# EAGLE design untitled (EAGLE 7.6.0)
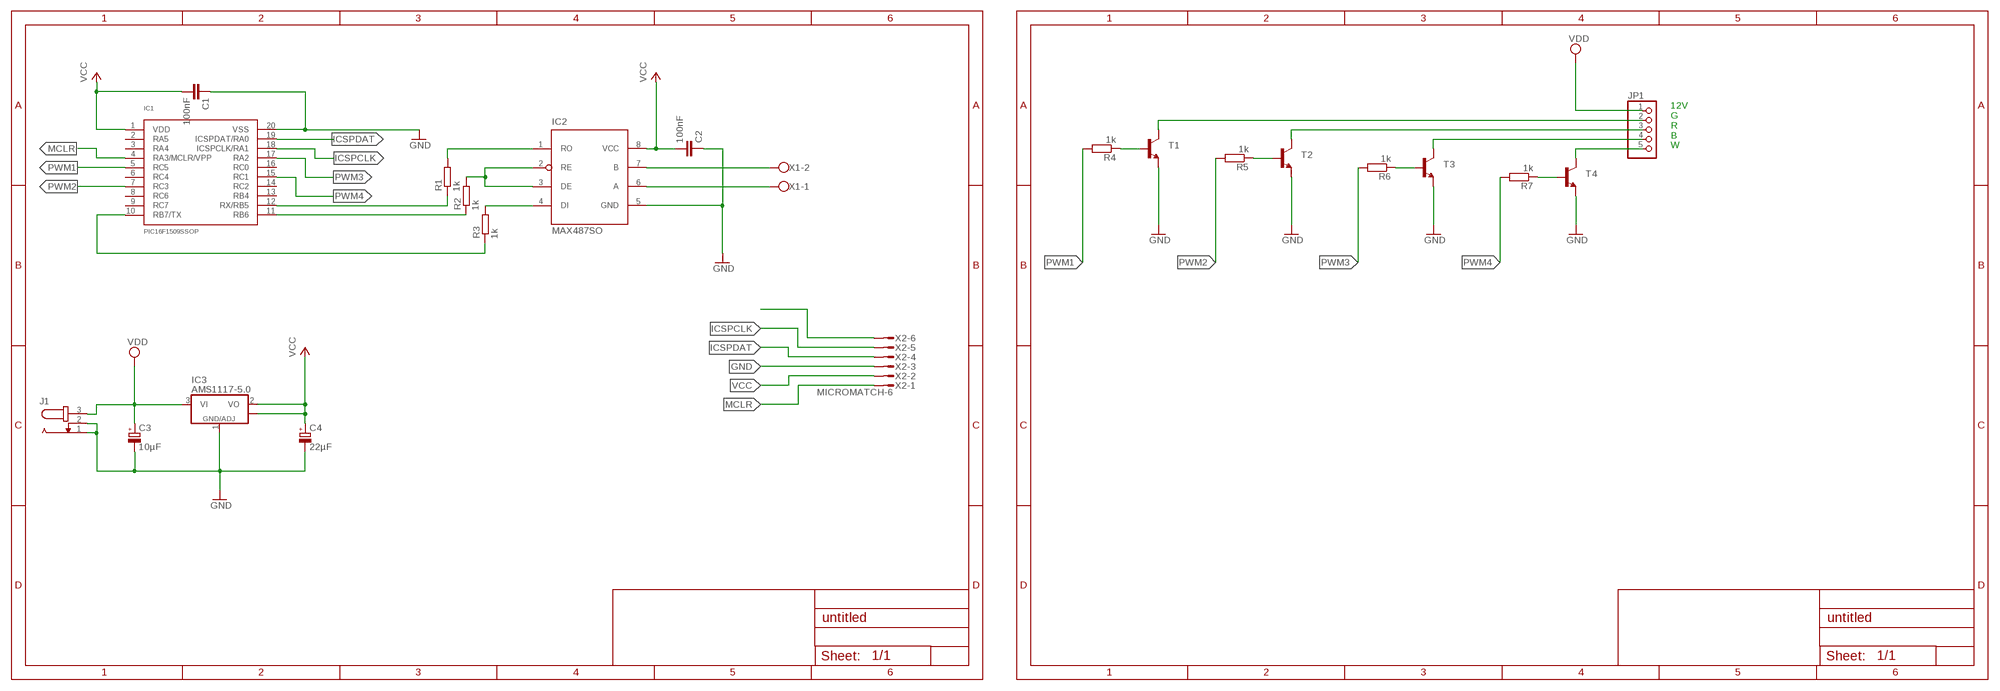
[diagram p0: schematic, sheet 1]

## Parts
C1  100nF  C-EUC0603  [C0603]
C2  100nF  C-EUC0603  [C0603]
C3  10µF  CPOL-EUF  [PANASONIC_F]
C4  22µF  CPOL-EUF  [PANASONIC_F]
IC1  PIC16F1509SSOP  [SSOP20]
IC2  MAX487SO  [SO08]
IC3  AMS1117-5.0  [SOT223]
J1  JACK-PLUG0  [SPC4077]
JP1  PINHD-1X5/90  [1X05/90]
R1  1k  R-EU_R0603  [R0603]
R2  1k  R-EU_R0603  [R0603]
R3  1k  R-EU_R0603  [R0603]
R4  1k  R-EU_R0603  [R0603]
R5  1k  R-EU_R0603  [R0603]
R6  1k  R-EU_R0603  [R0603]
R7  1k  R-EU_R0603  [R0603]
T1  -NPN-TO220V  [TO220V]
T2  -NPN-TO220V  [TO220V]
T3  -NPN-TO220V  [TO220V]
T4  -NPN-TO220V  [TO220V]
X1  W237-102  [W237-102]
X2  MICROMATCH-6  [MICROMATCH-6]

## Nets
GND: C1.1 C2.1 C3.- C4.- IC1.20(VSS) IC2.5(GND) IC3.1(GND/ADJ) J1.1 J1.2 T1.3(E) T2.3(E) T3.3(E) T4.3(E) X2.3
ICSPCLK: IC1.18(ICSPCLK/RA1) X2.5
ICSPDAT: IC1.19(ICSPDAT/RA0) X2.4
MCLR: IC1.4(RA3/MCLR/VPP) X2.1
N$1: JP1.2 T1.2(C)
N$2: IC1.10(RB7/TX) R3.1
N$3: IC2.2(RE) IC2.3(DE) R2.2
N$4: IC2.1(RO) R1.2
N$5: JP1.3 T2.2(C)
N$6: IC1.11(RB6) R2.1
N$7: IC1.12(RX/RB5) R1.1
N$8: IC2.4(DI) R3.2
N$9: JP1.4 T3.2(C)
N$10: JP1.5 T4.2(C)
N$11: IC2.7(B) X1.2
N$12: IC2.6(A) X1.1
N$13: R4.1 T1.1(B)
N$14: R5.1 T2.1(B)
N$15: R6.1 T3.1(B)
N$16: R7.1 T4.1(B)
N$22: X2.6
PWM1: IC1.5(RC5) R4.2
PWM2: IC1.7(RC3) R5.2
PWM3: IC1.17(RA2) R6.2
PWM4: IC1.15(RC1) R7.2
VCC: C1.2 C2.2 C4.+ IC1.1(VDD) IC2.8(VCC) IC3.2(VO) IC3.4(VO$1) X2.2
VDD: C3.+ IC3.3(VI) J1.3 JP1.1
Unconnected: IC1.2(RA5) IC1.3(RA4) IC1.6(RC4) IC1.8(RC6) IC1.9(RC7) IC1.13(RB4) IC1.14(RC2) IC1.16(RC0)

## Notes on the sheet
- 12V
  G
  R
  B
  W

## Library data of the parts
C1 C2 = rcl:C-EU: CAPACITOR, European symbol
C3 C4 = rcl:CPOL-EU: POLARIZED CAPACITOR, European symbol
IC1 = PIC16F:PIC16F1509: PIC16F1509 Flash: 14 KB RAM: 512 Byte Interner Oszillator: 16 MHz AD-Wandler: 12x 10-bit Schnittstellen: 1x UART, 1x SPI, 1x I2C Timer: 2x 8-bit, 1x 16-bit Besonderheiten: 4x 10-bit Standard-PWM
IC2 = maxim:MAX487
IC3 = AMS1117:AMS1117: Spannungsregler 1A
J1 = con-jack:JACK-PLUG: DC POWER JACK Power Jack, DC, Right Angle, Through Hole, Rated 5A at 16VDC, PC Terminals Distributor: Farnell (www.Farnell.de) Drawing: 84N1161.pdf / 84N1162.pdf Manufacturer: SPC Technology (www.spctechnology.com) Type: SPC4077 / SPC 4078; OC_FARNELL: unknown; OC_NEWARK: unknown
JP1 = pinhead:PINHD-1X5: PIN HEADER
R1-R7 = rcl:R-EU_: RESISTOR, European symbol
T1-T4 = transistor-neu-to92:*-NPN-: NPN Transistror
X1 = con-wago-500:W237-102: WAGO SCREW CLAMP; MPN: 237-102; OC_FARNELL: unknown; OC_NEWARK: 70K9898
X2 = con-amp-micromatch:MICROMATCH-6: MicroMaTch 6 7-215464-6 / 0-215464-6 Drawing Number C-215464 DDEController.pdf; MPN: 7-215464-6; OC_FARNELL: 3784630; OC_NEWARK: 19R8125

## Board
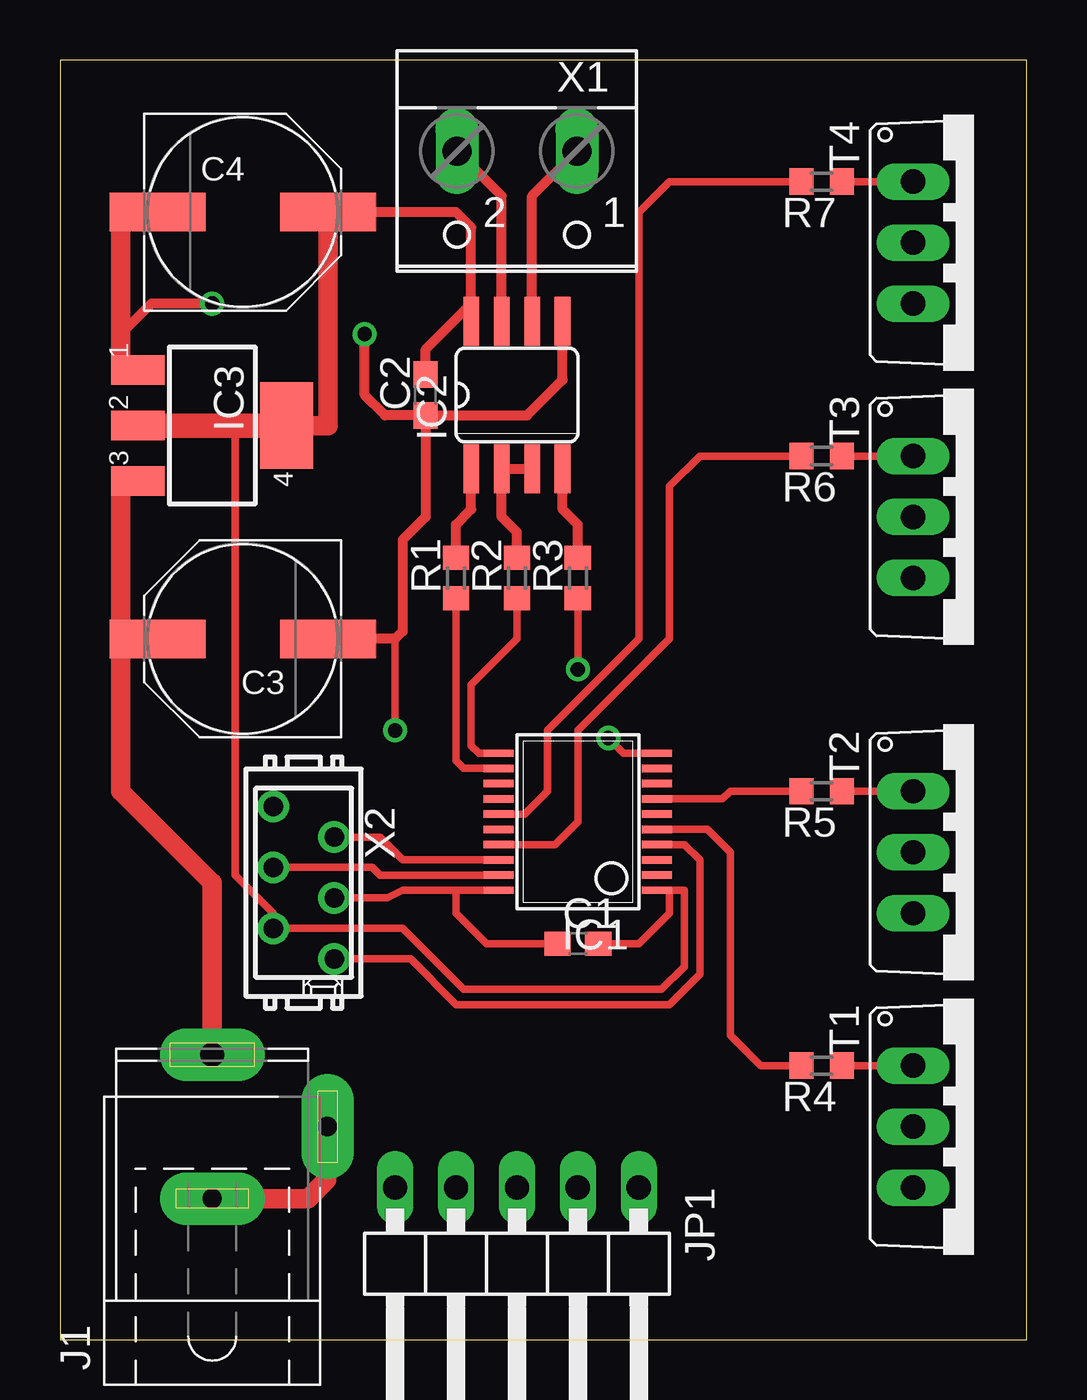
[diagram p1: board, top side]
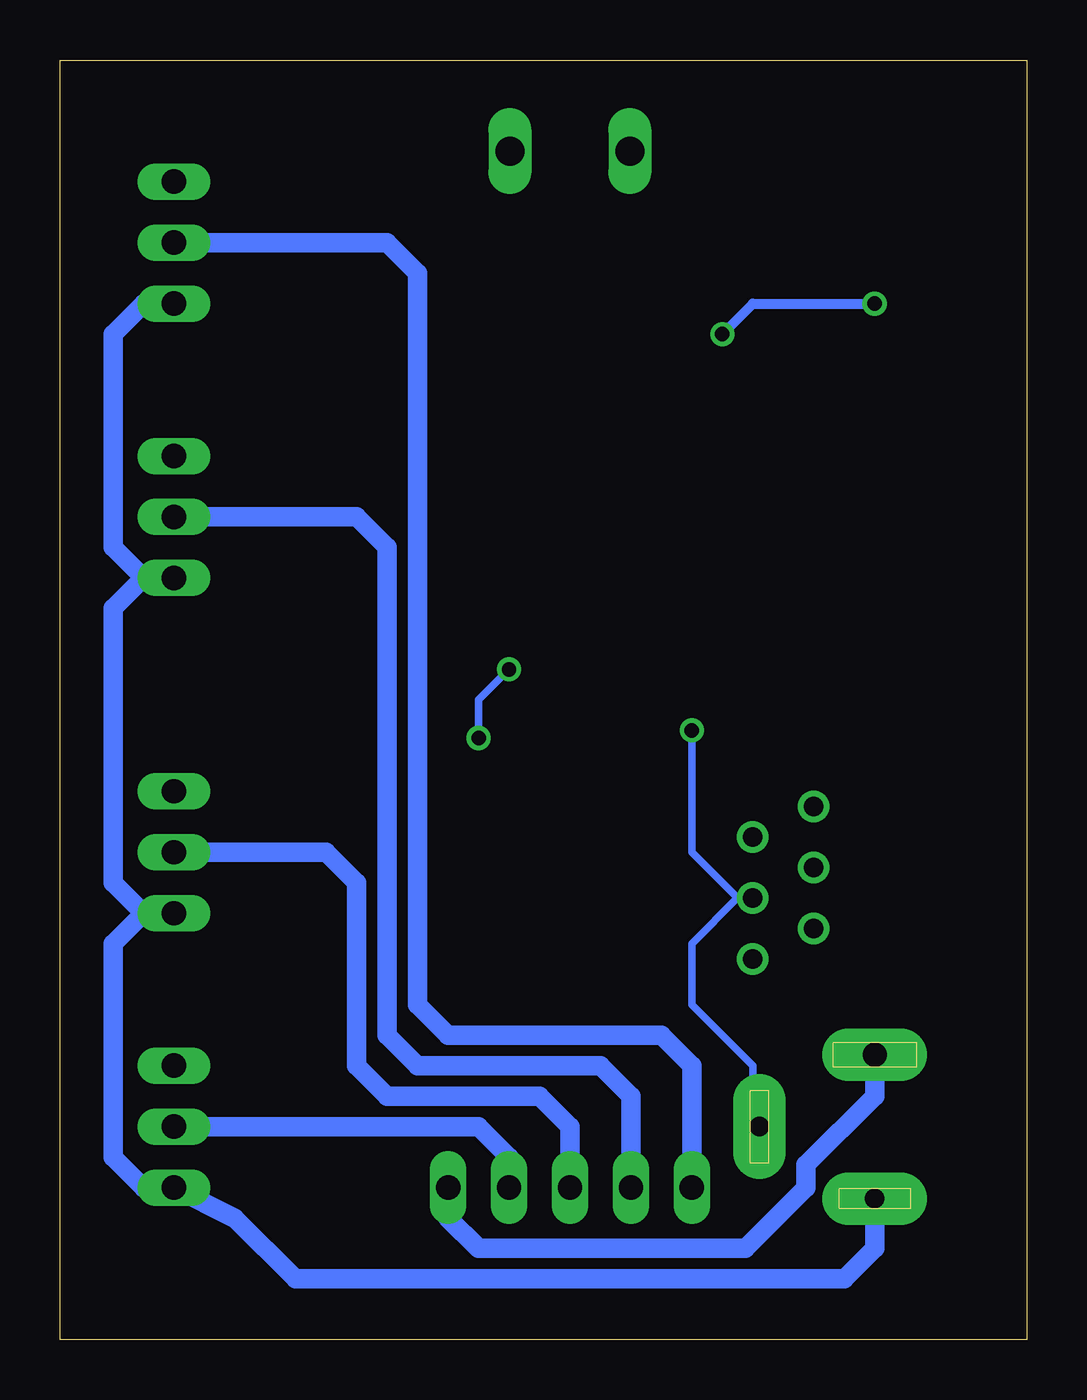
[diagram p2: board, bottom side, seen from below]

Size 40.31 x 53.33 mm. Coordinates in mm from the lower left corner, seen from the top.
Outline: 0,0 40.31,0 40.31,53.33 0,53.33 0,0
Copper layers (1*16): Top 0.035mm / dielectric 1.5mm / Bottom 0.035mm
Design rules "default": minimum track width 10mil, minimum drill 24mil, track to track 8mil, track to pad 8mil, pad to pad 8mil, via to via 8mil, smd to smd 8mil, copper to edge 40mil, drill to drill 8mil, minimum pad ring 10mil, minimum via ring 8mil, stop-mask expansion 4mil, vias tented up to drill 0mil, thermal gap 10mil

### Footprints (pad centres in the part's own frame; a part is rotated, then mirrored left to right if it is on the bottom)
C0603 = smd 1.1 x 1: 1 -0.85,0; 2 0.85,0
PANASONIC_F = smd 4 x 1.6: + 3.55,0; - -3.55,0
SSOP20 = smd 0.305 x 1.245: 1 -2.857,-3.302; 2 -2.222,-3.302; 3 -1.587,-3.302; 4 -0.952,-3.302; 5 -0.317,-3.302; 6 0.318,-3.302; 7 0.953,-3.302; 8 1.588,-3.302; 9 2.223,-3.302; 10 2.858,-3.302; 11 2.858,3.302; 12 2.223,3.302; 13 1.588,3.302; 14 0.953,3.302; 15 0.318,3.302; 16 -0.317,3.302; 17 -0.952,3.302; 18 -1.587,3.302; 19 -2.222,3.302; 20 -2.857,3.302
SO08 = smd 0.66 x 2.032: 1 -1.905,-3.073; 2 -0.635,-3.073; 3 0.635,-3.073; 4 1.905,-3.073; 5 1.905,3.073; 6 0.635,3.073; 7 -0.635,3.073; 8 -1.905,3.073
SOT223 = smd 1.219 x 2.235: 1 -2.311,-3.099; 2 0,-3.099; 3 2.311,-3.099 | smd 3.6 x 2.2: 4 0,3.099
SPC4077 = drill 0.8 pad 2.184 long: 1 -3,0; 2 0,-4.8 | drill 1 pad 2.184 long: 3 3,0
1X05/90 = drill 1.016 long: 1 -5.08,-3.81; 2 -2.54,-3.81; 3 0,-3.81; 4 2.54,-3.81; 5 5.08,-3.81
R0603 = smd 1 x 1.1: 1 -0.85,0; 2 0.85,0
TO220V = drill 1.016 long: 1 -2.54,-2.54; 2 0,-2.54; 3 2.54,-2.54
W237-102 = drill 1.194 long: 1 -2.5,-1.27; 2 2.5,-1.27
MICROMATCH-6 = drill 0.813: 1 3.175,1.27; 2 1.905,-1.27; 3 0.635,1.27; 4 -0.635,-1.27; 5 -1.905,1.27; 6 -3.175,-1.27

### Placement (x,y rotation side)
C1  21.59,16.51 0 top
C2  15.24,39.37 90 top
C3  7.62,29.21 180 top
C4  7.62,46.99 0 top
IC1  21.59,21.59 90 top
IC2  19.05,39.37 0 top
IC3  6.35,38.1 270 top
J1  6.35,8.89 90 top
JP1  19.05,2.54 180 top
R1  16.51,31.75 90 top
R2  19.05,31.75 90 top
R3  21.59,31.75 90 top
R4  31.75,11.43 180 top
R5  31.75,22.86 180 top
R6  31.75,36.83 180 top
R7  31.75,48.26 180 top
T1  38.1,8.89 270 top
T2  38.1,20.32 270 top
T3  38.1,34.29 270 top
T4  38.1,45.72 270 top
X1  19.05,48.26 180 top
X2  10.16,19.05 270 top

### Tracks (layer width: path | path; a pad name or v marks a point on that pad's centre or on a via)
GND  (via drill 0.6)
  Top 0.305: IC1.20 16.51,18.73 | 16.51,18.73 14.29,18.73 13.65,18.41 X2.3 | C1.1 17.78,16.51 16.51,17.78 16.51,18.73 | v13.97,25.4 13.97,29.21
  Top 0.406: C2.1 19.47,38.52 20.95,40.01 IC2.5 | C2.1 15.24,34.29 14.29,33.34 14.29,29.53 13.97,29.21 C3.- | C2.1 13.55,38.52 12.7,39.37 v12.7,41.91 | v6.35,43.18 3.81,43.18 2.54,41.91
  Top 0.813: J1.1 10.34,5.89 11.11,6.67 11.11,8.85 J1.2 | IC3.1 2.54,40.41 2.54,41.91 2.54,46.99 C4.-
  Bottom 0.305: 12.06,18.41 13.97,20.32 v13.97,25.4 | X2.3 12.06,18.41 | 12.06,18.41 13.97,16.51 13.97,13.97 11.43,11.43 11.43,9.17 J1.2
  Bottom 0.406: v12.7,41.91 11.43,43.18 v6.35,43.18
  Bottom 0.813: J1.1 6.35,3.81 7.62,2.54 30.48,2.54 33.02,5.08 T1.3 36.83,6.35 38.1,7.62 38.1,16.51 36.83,17.78 | T2.3 36.83,17.78 | 36.83,17.78 38.1,19.05 38.1,30.48 36.83,31.75 | T3.3 36.83,31.75 | 36.83,31.75 38.1,33.02 38.1,41.91 36.83,43.18 T4.3
ICSPCLK
  Top 0.305: IC1.18 14.29,20 13.34,20.95 X2.5
ICSPDAT
  Top 0.305: IC1.19 13.34,19.37 13.02,19.68 X2.4
MCLR
  Top 0.305: X2.1 14.61,15.88 16.51,13.97 25.4,13.97 26.67,15.24 26.67,20 26.04,20.64 IC1.4
N$1
  Bottom 0.813: T1.2 22.86,8.89 21.59,7.62 JP1.2
N$2  (via drill 0.6)
  Top 0.305: IC1.10 23.49,24.45 v22.86,25.08 | v21.59,27.94 R3.1
  Bottom 0.305: v22.86,25.08 22.86,26.67 v21.59,27.94
N$3
  Top 0.406: R2.2 19.05,33.66 18.41,34.29 IC2.2 IC2.3
N$4
  Top 0.406: R1.2 16.51,33.97 17.14,34.61 IC2.1
N$5
  Bottom 0.813: T2.2 29.21,20.32 27.94,19.05 27.94,11.43 26.67,10.16 20.32,10.16 19.05,8.89 JP1.3
N$6
  Top 0.305: IC1.11 17.46,24.45 17.14,24.77 17.14,27.3 19.05,29.21 R2.1
N$7
  Top 0.305: IC1.12 16.83,23.81 16.51,24.13 R1.1
N$8
  Top 0.406: R3.2 21.59,33.97 20.95,34.61 IC2.4
N$9
  Bottom 0.813: T3.2 27.94,34.29 26.67,33.02 26.67,12.7 25.4,11.43 17.78,11.43 16.51,10.16 JP1.4
N$10
  Bottom 0.813: T4.2 26.67,45.72 25.4,44.45 25.4,13.97 24.13,12.7 15.24,12.7 13.97,11.43 JP1.5
N$11
  Top 0.406: IC2.7 18.41,47.66 X1.2
N$12
  Top 0.406: IC2.6 19.68,47.66 X1.1
N$13
  Top 0.305: R4.1 T1.1
N$14
  Top 0.305: R5.1 T2.1
N$15
  Top 0.305: R6.1 T3.1
N$16
  Top 0.305: R7.1 T4.1
PWM1
  Top 0.305: IC1.5 26.99,21.27 27.94,20.32 27.94,12.7 29.21,11.43 R4.2
PWM2
  Top 0.305: IC1.7 27.62,22.54 27.94,22.86 R5.2
PWM3
  Top 0.305: R6.2 26.67,36.83 25.4,35.56 25.4,29.21 21.59,25.4 21.59,21.59 20.64,20.64 IC1.17
PWM4
  Top 0.305: IC1.15 19.37,21.91 20.32,22.86 20.32,25.4 24.13,29.21 24.13,46.99 25.4,48.26 R7.2
VCC
  Top 0.305: 25.4,18.73 26.04,18.73 26.04,15.56 25.08,14.61 16.83,14.61 14.29,17.14 X2.2 8.89,17.78 7.3,19.37 7.3,37.78 7.62,38.1 | 25.4,18.73 IC1.1 | IC1.1 | C1.2 24.13,16.51 25.4,17.78 25.4,18.73
  Top 0.406: IC2.8 17.14,43.18 | 17.14,43.18 17.14,46.35 16.51,46.99 C4.+ | C2.2 15.24,41.27 17.14,43.18
  Top 0.813: IC3.4 11.17,38.1 C4.+
  Top 1.016: IC3.2 7.62,38.1 IC3.4
VDD
  Top 0.813: IC3.3 2.54,35.79 2.54,29.21 | 2.54,29.21 C3.+ | J1.3 6.35,19.05 2.54,22.86 2.54,29.21
  Bottom 0.813: JP1.1 24.13,5.08 22.86,3.81 11.75,3.81 9.21,6.35 9.21,7.3 6.35,10.16 J1.3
